(* Logix 5000 DataType export wxsGlobalControl; software revision 32.00 *)

TYPE wxsGlobalControl :   // Revolution St. WXS UDT
STRUCT
   GlobalStart : wxsPushbutton;   // Global Start
   GlobalStop : wxsPushbutton;   // Global Stop
   GlobalReset : wxsPushbutton;   // Global Reset
   GlobalEmergencyStop : wxsPushbutton;   // Emergency Stop
   GlobalStatus : STRING;   // Global System Status
   GlobalShiftActive : BOOL;   // Shift Active
END_STRUCT
END_TYPE

TYPE wxsPushbutton :
STRUCT
   Active : BOOL;   // Mouse Click
   Enable : BOOL;   // Enable/Disable
END_STRUCT
END_TYPE
